| TEXAS INSTRUMENTS INCORPORATED
| Standard Linear and Logic Group
| IBIS Model of SN74LVTH162245
| 3.3-V ABT 16-BIT BUS TRANSCEIVERS WITH 3-STATE OUTPUTS
| This file contains package information for the following:
|  TSSOP 48-pin (DGG) package as [Component] LVTH162245_DGG
|  SSOP 48-pin (DL) package as [Component] LVTH162245_DL
|  U*BGA 48-pin (GQL) package as [Component] LVTH162245_GQL
| This device can be powered at the following Vccs:
|  2.7 volt Vcc
|  3.3 volt Vcc
| This file provides unique models under the [Model Selector] for each Vcc.
| For operation at a specific Vcc, select the appropriate model after each
| [Model Selector] keyword.
[IBIS Ver]   3.2
[Comment char]  |_char
[File Name]   sn74lvth162245.ibs
[File Rev]   1.1 | b_die
[Date]   March 27, 2003
[Source]   Data created from TI-SPICE simulations at TI-SLL.
[Notes]   The following is an IBIS list for the LVTH162245.
   Please contact sllibis@ti.com with questions and
   comments concerning SLL IBIS models.
   - Power-clamp data has been deleted since there is no
   power-clamp diode in the device.
   - Due to presence of bus hold at input, GND-clamp curves
   have non-monotonic warnings.
   - Non-monotonic data in pullup/pulldown data due to damping
   resistor.
[Disclaimer] Property of Texas Instruments Incorporated.  Unauthorized
   reproduction and/or distribution is strictly prohibited.
   This product is protected under copyright law.
   Created  2003, (C) Copyright  2003, Texas Instruments
   Incorporated, All Rights Reserved
   UNLESS THERE IS A SIGNED, WRITTEN AGREEMENT TO THE
   CONTRARY, TEXAS INSTRUMENTS (TI) IS PROVIDING THE IBIS
   MODELS  AND WITHOUT ANY WARRANTY, EXPRESSED OR
   IMPLIED.  TI assumes no liability for:
   1) the accuracy of the IBIS models provided to your
   company;
   2) the proper functioning of these IBIS Models in your
   design or for any resulting applications; or
   3) infringement of patents, copyrights or intellectual
   property rights resulting from your use of these IBIS
   models.
   TI provides IBIS Models as a service to our customers.
   You and your company shall not distribute, sell or give
   these models to anyone else without prior written
   permission from TI.
   TI reserves the right to make changes to our products or
   to discontinue any semiconductor product or service
   without notice, and advises our customers to obtain the
   latest version of relevant information to verify, before
   placing orders, that the information being relied on is
   current.
   Please be aware that your receipt and use of the IBIS
   information provided shall serve as acceptance of these
   terms and conditions.  If you do not accept these terms,
   you should return or destroy the IBIS models and any
   other accompanying information immediately.
| Component LVTH162245_DGG 48-pin TSSOP
[Component]   LVTH162245_DGG
[Manufacturer]   Texas Instruments, Inc.
[Package]
|   typ   min   max
R_pkg   4.400e-02   3.800e-02   5.100e-02
L_pkg   3.019e-09   2.486e-09   4.099e-09
C_pkg   5.070e-13   3.340e-13   8.090e-13
[Pin]   signal_name   model_name   R_pin   L_pin   C_pin
1   1DIR   LVTH162245_DIR   4.100e-02   4.017e-09   7.590e-13
2   1B1   LVTH162245_BIO   4.200e-02   3.737e-09   7.920e-13
3   1B2   LVTH162245_BIO   4.200e-02   3.480e-09   6.610e-13
4   GND   GND   3.800e-02   3.131e-09   5.750e-13
5   1B3   LVTH162245_BIO   4.700e-02   3.122e-09   5.660e-13
6   1B4   LVTH162245_BIO   4.300e-02   2.948e-09   5.040e-13
7   VCC   POWER   4.500e-02   2.845e-09   3.970e-13
8   1B5   LVTH162245_BIO   4.900e-02   2.835e-09   3.940e-13
9   1B6   LVTH162245_BIO   4.800e-02   2.715e-09   3.780e-13
10   GND   GND   5.000e-02   2.664e-09   3.630e-13
11   1B7   LVTH162245_BIO   5.000e-02   2.585e-09   3.480e-13
12   1B8   LVTH162245_BIO   4.900e-02   2.550e-09   3.370e-13
13   2B1   LVTH162245_BIO   4.900e-02   2.541e-09   3.360e-13
14   2B2   LVTH162245_BIO   5.000e-02   2.574e-09   3.480e-13
15   GND   GND   4.900e-02   2.618e-09   3.590e-13
16   2B3   LVTH162245_BIO   4.600e-02   2.671e-09   3.750e-13
17   2B4   LVTH162245_BIO   4.500e-02   2.754e-09   3.890e-13
18   VCC   POWER   4.400e-02   2.823e-09   4.500e-13
19   2B5   LVTH162245_BIO   4.200e-02   2.968e-09   5.030e-13
20   2B6   LVTH162245_BIO   5.100e-02   3.108e-09   5.350e-13
21   GND   GND   4.200e-02   3.175e-09   5.870e-13
22   2B7   LVTH162245_BIO   4.100e-02   3.449e-09   6.780e-13
23   2B8   LVTH162245_BIO   4.400e-02   3.766e-09   8.040e-13
24   2DIR   LVTH162245_DIR   4.300e-02   4.065e-09   7.610e-13
25   2NOE   LVTH162245_OE   4.100e-02   3.994e-09   7.570e-13
26   2A8   LVTH162245_AIO   3.900e-02   3.649e-09   7.890e-13
27   2A7   LVTH162245_AIO   3.800e-02   3.362e-09   6.600e-13
28   GND   GND   3.800e-02   3.082e-09   5.740e-13
29   2A6   LVTH162245_AIO   4.400e-02   2.990e-09   5.220e-13
30   2A5   LVTH162245_AIO   4.100e-02   2.917e-09   4.950e-13
31   VCC   POWER   4.300e-02   2.820e-09   4.480e-13
32   2A4   LVTH162245_AIO   4.300e-02   2.699e-09   3.850e-13
33   2A3   LVTH162245_AIO   4.500e-02   2.628e-09   3.720e-13
34   GND   GND   4.600e-02   2.556e-09   3.560e-13
35   2A2   LVTH162245_AIO   4.600e-02   2.495e-09   3.440e-13
36   2A1   LVTH162245_AIO   4.700e-02   2.487e-09   3.340e-13
37   1A8   LVTH162245_AIO   4.700e-02   2.490e-09   3.350e-13
38   1A7   LVTH162245_AIO   4.600e-02   2.486e-09   3.430e-13
39   GND   GND   4.500e-02   2.566e-09   3.560e-13
40   1A6   LVTH162245_AIO   4.400e-02   2.639e-09   3.740e-13
41   1A5   LVTH162245_AIO   4.300e-02   2.701e-09   3.860e-13
42   VCC   POWER   4.300e-02   2.817e-09   4.500e-13
43   1A4   LVTH162245_AIO   4.100e-02   2.935e-09   5.010e-13
44   1A3   LVTH162245_AIO   4.700e-02   3.035e-09   5.290e-13
45   GND   GND   4.300e-02   3.171e-09   5.890e-13
46   1A2   LVTH162245_AIO   4.000e-02   3.415e-09   6.820e-13
47   1A1   LVTH162245_AIO   4.300e-02   3.741e-09   8.090e-13
48   1NOE   LVTH162245_OE   4.400e-02   4.099e-09   7.640e-13
| Component LVTH162245_DL 48-pin SSOP
[Component]   LVTH162245_DL
[Manufacturer]   Texas Instruments, Inc.
[Package]
|   typ   min   max
R_pkg   4.800e-02   3.800e-02   5.300e-02
L_pkg   6.046e-09   5.084e-09   7.968e-09
C_pkg   8.130e-13   5.690e-13   1.157e-12
[Pin]   signal_name   model_name   R_pin   L_pin   C_pin
1   1DIR   LVTH162245_DIR   4.600e-02   7.968e-09   1.017e-12
2   1B1   LVTH162245_BIO   4.400e-02   7.299e-09   1.157e-12
3   1B2   LVTH162245_BIO   4.300e-02   6.765e-09   1.058e-12
4   GND   GND   4.100e-02   6.269e-09   9.330e-13
5   1B3   LVTH162245_BIO   3.800e-02   5.856e-09   8.290e-13
6   1B4   LVTH162245_BIO   4.600e-02   5.802e-09   7.900e-13
7   VCC   POWER   5.000e-02   5.656e-09   7.380e-13
8   1B5   LVTH162245_BIO   5.300e-02   5.500e-09   6.430e-13
9   1B6   LVTH162245_BIO   5.200e-02   5.304e-09   6.060e-13
10   GND   GND   5.300e-02   5.189e-09   5.830e-13
11   1B7   LVTH162245_BIO   5.100e-02   5.084e-09   5.690e-13
12   1B8   LVTH162245_BIO   5.300e-02   5.862e-09   8.330e-13
13   2B1   LVTH162245_BIO   5.300e-02   5.862e-09   8.330e-13
14   2B2   LVTH162245_BIO   5.100e-02   5.084e-09   5.690e-13
15   GND   GND   5.300e-02   5.189e-09   5.830e-13
16   2B3   LVTH162245_BIO   5.200e-02   5.304e-09   6.060e-13
17   2B4   LVTH162245_BIO   5.300e-02   5.500e-09   6.430e-13
18   VCC   POWER   5.000e-02   5.656e-09   7.380e-13
19   2B5   LVTH162245_BIO   4.600e-02   5.802e-09   7.900e-13
20   2B6   LVTH162245_BIO   3.800e-02   5.856e-09   8.290e-13
21   GND   GND   4.100e-02   6.269e-09   9.330e-13
22   2B7   LVTH162245_BIO   4.300e-02   6.765e-09   1.058e-12
23   2B8   LVTH162245_BIO   4.400e-02   7.299e-09   1.157e-12
24   2DIR   LVTH162245_DIR   4.600e-02   7.968e-09   1.017e-12
25   2NOE   LVTH162245_OE   4.600e-02   7.968e-09   1.017e-12
26   2A8   LVTH162245_AIO   4.400e-02   7.299e-09   1.157e-12
27   2A7   LVTH162245_AIO   4.300e-02   6.765e-09   1.058e-12
28   GND   GND   4.100e-02   6.269e-09   9.330e-13
29   2A6   LVTH162245_AIO   3.800e-02   5.856e-09   8.290e-13
30   2A5   LVTH162245_AIO   4.600e-02   5.802e-09   7.900e-13
31   VCC   POWER   5.000e-02   5.656e-09   7.380e-13
32   2A4   LVTH162245_AIO   5.300e-02   5.500e-09   6.430e-13
33   2A3   LVTH162245_AIO   5.200e-02   5.304e-09   6.060e-13
34   GND   GND   5.300e-02   5.189e-09   5.830e-13
35   2A2   LVTH162245_AIO   5.100e-02   5.084e-09   5.690e-13
36   2A1   LVTH162245_AIO   5.300e-02   5.862e-09   8.330e-13
37   1A8   LVTH162245_AIO   5.300e-02   5.862e-09   8.330e-13
38   1A7   LVTH162245_AIO   5.100e-02   5.084e-09   5.690e-13
39   GND   GND   5.300e-02   5.189e-09   5.830e-13
40   1A6   LVTH162245_AIO   5.200e-02   5.304e-09   6.060e-13
41   1A5   LVTH162245_AIO   5.300e-02   5.500e-09   6.430e-13
42   VCC   POWER   5.000e-02   5.656e-09   7.380e-13
43   1A4   LVTH162245_AIO   4.600e-02   5.802e-09   7.900e-13
44   1A3   LVTH162245_AIO   3.800e-02   5.856e-09   8.290e-13
45   GND   GND   4.100e-02   6.269e-09   9.330e-13
46   1A2   LVTH162245_AIO   4.300e-02   6.765e-09   1.058e-12
47   1A1   LVTH162245_AIO   4.400e-02   7.299e-09   1.157e-12
48   1NOE   LVTH162245_OE   4.600e-02   7.967e-09   1.017e-12
| Component LVTH162245_GQL 48-pin U*BGA
[Component]   LVTH162245_GQL
[Manufacturer]   Texas Instruments, Inc.
[Package]
|   typ   min   max
R_pkg   7.900e-02   4.500e-02   9.400e-02
L_pkg   2.264e-09   1.398e-09   2.722e-09
C_pkg   3.060e-13   1.170e-13   4.040e-13
[Pin]   signal_name   model_name   R_pin   L_pin   C_pin
A1   1DIR   LVTH162245_DIR   5.100e-02   1.531e-09   2.100e-13
B2   1B1   LVTH162245_BIO   7.300e-02   2.572e-09   3.120e-13
B1   1B2   LVTH162245_BIO   7.100e-02   1.835e-09   2.320e-13
B3   GND   GND   9.400e-02   2.717e-09   3.830e-13
C2   1B3   LVTH162245_BIO   8.900e-02   2.534e-09   3.500e-13
C1   1B4   LVTH162245_BIO   7.100e-02   1.831e-09   2.310e-13
C3   VCC   POWER   9.400e-02   2.722e-09   3.920e-13
D2   1B5   LVTH162245_BIO   9.000e-02   2.551e-09   3.520e-13
D1   1B6   LVTH162245_BIO   7.200e-02   1.846e-09   2.440e-13
D3   GND   GND   9.400e-02   2.719e-09   4.030e-13
E2   1B7   LVTH162245_BIO   8.900e-02   2.541e-09   3.510e-13
E1   1B8   LVTH162245_BIO   7.200e-02   1.850e-09   2.270e-13
F1   2B1   LVTH162245_BIO   7.200e-02   1.850e-09   2.270e-13
F2   2B2   LVTH162245_BIO   8.900e-02   2.541e-09   3.510e-13
G3   GND   GND   9.400e-02   2.718e-09   4.040e-13
G1   2B3   LVTH162245_BIO   7.200e-02   1.847e-09   2.440e-13
G2   2B4   LVTH162245_BIO   9.000e-02   2.551e-09   3.520e-13
H3   VCC   POWER   9.400e-02   2.721e-09   3.920e-13
H1   2B5   LVTH162245_BIO   7.000e-02   1.830e-09   2.310e-13
H2   2B6   LVTH162245_BIO   8.800e-02   2.524e-09   3.500e-13
J3   GND   GND   9.300e-02   2.709e-09   3.820e-13
J1   2B7   LVTH162245_BIO   7.100e-02   1.851e-09   2.330e-13
J2   2B8   LVTH162245_BIO   5.600e-02   2.605e-09   3.900e-13
K1   2DIR   LVTH162245_DIR   4.500e-02   1.398e-09   1.170e-13
K6   2NOE   LVTH162245_OE   4.500e-02   1.512e-09   1.930e-13
J5   2A8   LVTH162245_AIO   5.500e-02   2.492e-09   3.130e-13
J6   2A7   LVTH162245_AIO   7.000e-02   1.821e-09   2.300e-13
J4   GND   GND   9.300e-02   2.703e-09   3.820e-13
H5   2A6   LVTH162245_AIO   8.900e-02   2.529e-09   3.500e-13
H6   2A5   LVTH162245_AIO   7.100e-02   1.826e-09   2.300e-13
H4   VCC   POWER   9.400e-02   2.722e-09   3.910e-13
G5   2A4   LVTH162245_AIO   9.000e-02   2.551e-09   3.520e-13
G6   2A3   LVTH162245_AIO   7.200e-02   1.846e-09   2.440e-13
G4   GND   GND   9.400e-02   2.719e-09   4.040e-13
F5   2A2   LVTH162245_AIO   8.800e-02   2.510e-09   3.490e-13
F6   2A1   LVTH162245_AIO   7.200e-02   1.850e-09   2.270e-13
E6   1A8   LVTH162245_AIO   7.100e-02   1.850e-09   2.270e-13
E5   1A7   LVTH162245_AIO   8.900e-02   2.529e-09   3.500e-13
D4   GND   GND   9.400e-02   2.719e-09   4.030e-13
D6   1A6   LVTH162245_AIO   7.200e-02   1.847e-09   2.430e-13
D5   1A5   LVTH162245_AIO   8.900e-02   2.550e-09   3.520e-13
C4   VCC   POWER   9.400e-02   2.722e-09   3.910e-13
C6   1A4   LVTH162245_AIO   7.100e-02   1.827e-09   2.300e-13
C5   1A3   LVTH162245_AIO   8.900e-02   2.539e-09   3.500e-13
B4   GND   GND   9.300e-02   2.705e-09   3.820e-13
B6   1A2   LVTH162245_AIO   7.100e-02   1.831e-09   2.270e-13
B5   1A1   LVTH162245_AIO   7.300e-02   2.685e-09   3.800e-13
A6   1NOE   LVTH162245_OE   5.100e-02   1.417e-09   1.330e-13
| Model LVTH162245_OE
[Model Selector]   LVTH162245_OE
LVTH162245_OE_27   2.7 volt Vcc
LVTH162245_OE_33   3.3 volt Vcc
| Model LVTH162245_DIR
[Model Selector]   LVTH162245_DIR
LVTH162245_DIR_27   2.7 volt Vcc
LVTH162245_DIR_33   3.3 volt Vcc
| Model LVTH162245_AIO
[Model Selector]   LVTH162245_AIO
LVTH162245_AIO_27   2.7 volt Vcc
LVTH162245_AIO_33   3.3 volt Vcc
| Model LVTH162245_BIO
[Model Selector]   LVTH162245_BIO
LVTH162245_BIO_27   2.7 volt Vcc
LVTH162245_BIO_33   3.3 volt Vcc
| Models and submodels in the file (8): LVTH162245_OE_27 (Input), LVTH162245_OE_33 (Input), LVTH162245_DIR_27 (Input), LVTH162245_DIR_33 (Input), LVTH162245_AIO_27 (I/O), LVTH162245_AIO_33 (I/O), LVTH162245_BIO_27 (I/O), LVTH162245_BIO_33 (I/O)
